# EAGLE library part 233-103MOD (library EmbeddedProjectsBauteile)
CON WAGO 255 3polig modifiziert
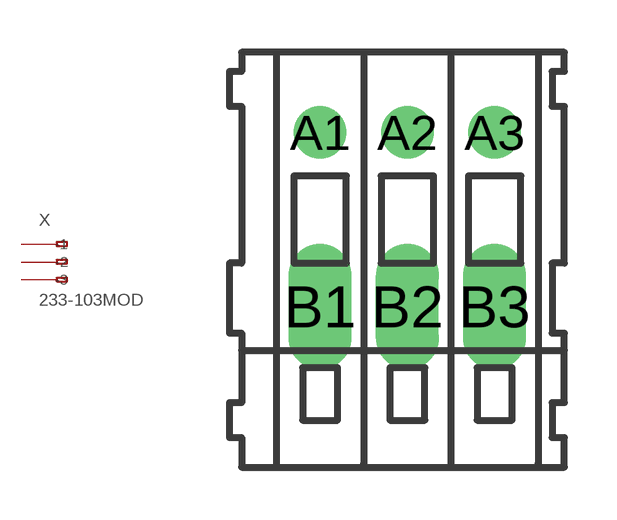
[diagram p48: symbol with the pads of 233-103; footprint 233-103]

Designator prefix X

## 233-103MOD  [233-103]
A1  -1  pas
A2  -2  pas
A3  -3  pas
B1  B-1  pas
B2  B-2  pas
B3  B-3  pas

## Footprint 233-103 (pad centres in mm)
WAGO
drill 1 pad 1.422: A1 -2.5,2.5; A2 0,2.5; A3 2.5,2.5
drill 1.2 long: B1 -2.5,-2.5; B2 0,-2.5; B3 2.5,-2.5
